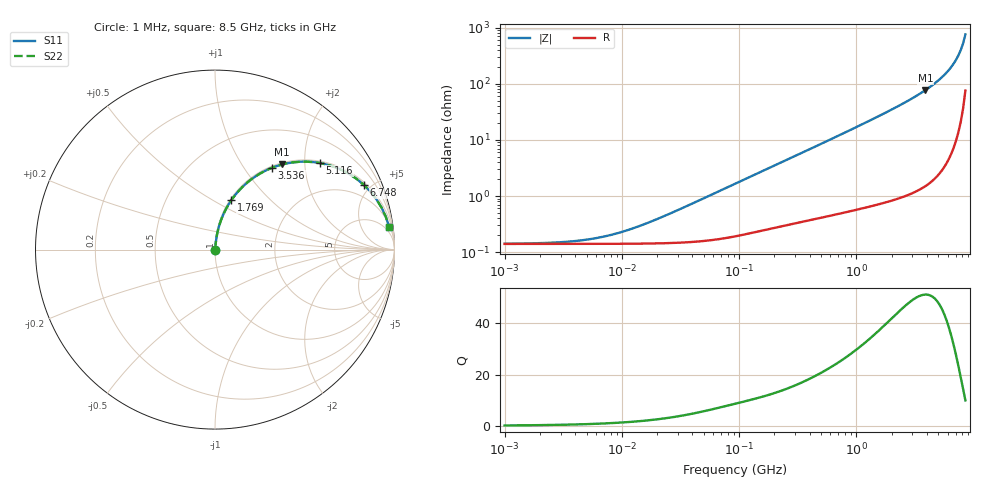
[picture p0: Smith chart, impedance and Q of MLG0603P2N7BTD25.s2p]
! S-Parameter Data Generated by TDK Corporation
! Copyright(C) 2025 TDK Corporation.
! All Rights Reserved.
! TDK P/N: MLG0603P2N7BTD25 (SMD / SMT Inductor (Coil))
! Property: L=2.7nH at 500MHz
! Size(LxWxT): 0.6x0.3x0.3mm
! Model Type: s2p (Touchstone File Format Version 1.0)
! Frequency: DC=Yes Start=1MHz Stop=8500MHz 198points Log-sweep
! Model Generated on Feb. 6, 2025
! Terms and conditions regarding TDK Simulation Models:
! 1)This simulation model is being provided solely for informational
!  purposes. Please refer to the specifications of the products in
!  terms of detailed characteristics of such products.
! 2)In no event shall TDK Corporation of any of its subsidiaries be
!  liable for any loss or damage arising, directly or indirectly,
!  from any information contained in this simulation model, including,
!  but not limited to loss or damages arising from any inaccuracies,
!  omissions or errors in connection with such information.
! 3)Any and all copyrights on this simulation model are owned by
!  TDK Corporation.  Duplication or redistribution of this simulation
!  model without prior written permission from TDK Corporation
!  is prohibited.
! 4)This simulation model is subject to any modification or change
!  without any prior notice.
! 5)Neither TDK Corporation nor any of its subsidiaries shall make any
!  warranty, express or implied, including but not limited to the
!  correctness, implied warranties of merchantability and fitness for
!  a particular purpose with respect to this simulation models.
! 6)The use of this simulation model shall be deemed to have consented
!  to the terms and conditions hereof.
! Port Assignments:
!  1 ---@@@--- 2
! Applicable Conditions:
!  Temperature = 25 degC
!  DC Bias Current = 0 A
!  Small Signal Operation
# Hz S MA R 50
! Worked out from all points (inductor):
!   197 points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, 1 MHz to 8.5 GHz, reference 50 ohm
!   read as one part in series: L = 2.87 nH near 24.17 MHz
!   highest Q = 51.3 at 3.878 GHz (marker M1), where L = 3.16 nH
!   S11 on the Smith chart (normalised r, x): 1 MHz: 1.00, +0.00; 1.769 GHz: 1.02, +0.61; 3.536 GHz: 1.03, +1.36; 5.116 GHz: 1.05, +2.39; 6.748 GHz: 1.14, +4.56; 8.5 GHz: 3, +15
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1000000  0.00141 7.3  0.9986 -0.0  0.9986 -0.0  0.00141 7.3
2517452  0.001471 18.0  0.9986 -0.0  0.9986 -0.0  0.001471 18.0
4587603  0.001626 30.6  0.9986 -0.0  0.9986 -0.0  0.001626 30.6
6636977  0.001844 40.5  0.9986 -0.1  0.9986 -0.1  0.001844 40.5
9601846  0.002231 50.9  0.9986 -0.1  0.9986 -0.1  0.002231 50.9
1.389118e7  0.002877 60.4  0.9986 -0.1  0.9986 -0.1  0.002877 60.4
2.10461e7  0.004056 69.1  0.9986 -0.2  0.9986 -0.2  0.004056 69.1
9.219544e7  0.01646 82.4  0.998 -0.9  0.998 -0.9  0.01646 82.4
4.229561e8  0.07161 82.9  0.9937 -4.1  0.9937 -4.1  0.07161 82.9
9.270694e8  0.154 79.1  0.9827 -8.9  0.9827 -8.9  0.154 79.1
1.769233e9  0.289 71.8  0.9501 -16.8  0.9501 -16.8  0.289 71.8
1.940355e9  0.316 70.2  0.9411 -18.4  0.9411 -18.4  0.316 70.2
2.680511e9  0.4306 63.3  0.8935 -25.5  0.8935 -25.5  0.4306 63.3
3.535948e9  0.5565 55.1  0.82 -33.8  0.82 -33.8  0.5565 55.1
3.877948e9  0.6042 51.7  0.7852 -37.2  0.7852 -37.2  0.6042 51.7
5.115526e9  0.7589 39.4  0.6354 -49.3  0.6354 -49.3  0.7589 39.4
5.87536e9  0.8362 31.9  0.5284 -56.7  0.5284 -56.7  0.8362 31.9
6.748056e9  0.9054 23.4  0.3969 -64.8  0.3969 -64.8  0.9054 23.4
7.400733e9  0.9427 17.2  0.2961 -70.4  0.2961 -70.4  0.9427 17.2
7.750377e9  0.9576 14.0  0.2423 -73.0  0.2423 -73.0  0.9576 14.0
8.116539e9  0.9697 10.7  0.1867 -75.3  0.1867 -75.3  0.9697 10.7
8.5e9  0.9786 7.4  0.1297 -76.8  0.1297 -76.8  0.9786 7.4
